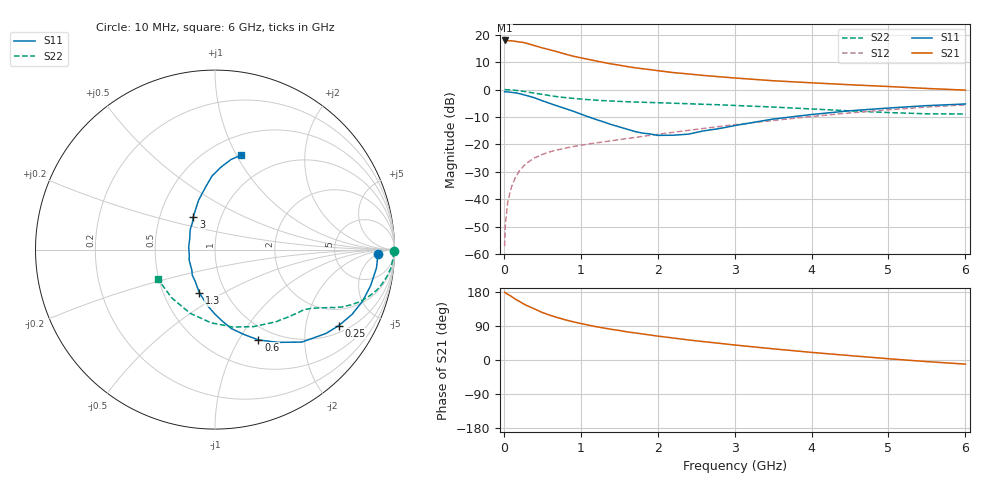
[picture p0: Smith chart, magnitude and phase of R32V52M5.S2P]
! SIEMENS Small Signal Semiconductors
! BFR181
! Si NPN RF Bipolar Junction Transistor in SOT23
! VCE = 2.5 V  IC = 2.5 mA
! Common Emitter S-Parameters:  May  1996
# GHz  S  MA  R  50
!  f  S11  S21  S12  S22
! GHz  MAG  ANG  MAG  ANG  MAG  ANG  MAG  ANG
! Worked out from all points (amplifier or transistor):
!   36 points, 10 MHz to 6 GHz, reference 50 ohm
!   highest |S21| = 17.9 dB at 10 MHz (marker M1)
!   |S21| within 3 dB of that: start of sweep to 541.2 MHz
!   unconditionally stable (mu >= 1): 1.437 GHz to 3.27 GHz
!   at 250 MHz: K = 0.27, MSG = 22.6 dB, |S12| = -28.1 dB
!   at 1.4 GHz: K = 0.99, MSG = 14.0 dB, |S12| = -18.7 dB
!   at 6 GHz: K = 0.86, MSG = 2.7 dB, |S12| = -5.6 dB
!   S11 on the Smith chart (normalised r, x): 10 MHz: 20, -5; 250 MHz: 1.25, -3.07; 600 MHz: 0.83, -1.22; 1.3 GHz: 0.75, -0.39; 3 GHz: 0.74, +0.29; 6 GHz: 0.70, +1.04
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0.01  0.9092 -1.4  7.843 178.9  0.0014 94.1  0.9964 -0.6
0.02  0.9073 -2.7  7.823 177.2  0.0034 89.3  0.9951 -1.3
0.05  0.9053 -6.5  7.76 173.7  0.0089 84.5  0.9928 -3.0
0.1  0.8902 -13.0  7.738 167.5  0.0169 82.7  0.9851 -6.1
0.15  0.871 -19.3  7.541 160.5  0.0249 78.2  0.9685 -9.1
0.25  0.8091 -31.6  7.219 148.9  0.0394 71.9  0.9298 -14.0
0.3  0.7748 -37.1  6.937 143.4  0.046 69.4  0.9045 -16.2
0.4  0.7067 -46.8  6.313 134.7  0.0569 65.0  0.8599 -19.7
0.5  0.625 -55.8  5.74 125.4  0.0658 61.8  0.8163 -22.2
0.6  0.5585 -64.3  5.295 118.1  0.0734 59.2  0.7743 -24.4
0.7  0.5003 -71.1  4.856 111.8  0.0798 57.8  0.7393 -25.9
0.8  0.4498 -78.2  4.417 106.0  0.0855 56.5  0.7121 -26.9
0.9  0.4035 -83.8  4.062 100.9  0.0915 55.8  0.6907 -28.0
1.1  0.3177 -97.1  3.544 92.1  0.1018 55.7  0.6549 -29.8
1.3  0.2562 -109.8  3.107 84.4  0.1118 55.9  0.6276 -31.4
1.6  0.1901 -131.8  2.627 74.3  0.1278 56.7  0.5999 -34.0
2.2  0.1471 174.0  2.038 58.1  0.1662 57.8  0.5634 -40.6
3  0.2203 123.2  1.624 39.6  0.2287 56.1  0.5131 -52.8
3.5  0.2899 108.4  1.447 29.5  0.2733 53.4  0.4799 -63.4
4.5  0.4107 92.3  1.223 11.6  0.3751 44.5  0.4084 -93.1
5.5  0.5093 80.0  1.046 -4.2  0.4791 31.8  0.3612 -131.8
6  0.5461 74.6  0.976 -10.9  0.526 24.6  0.3585 -152.8
